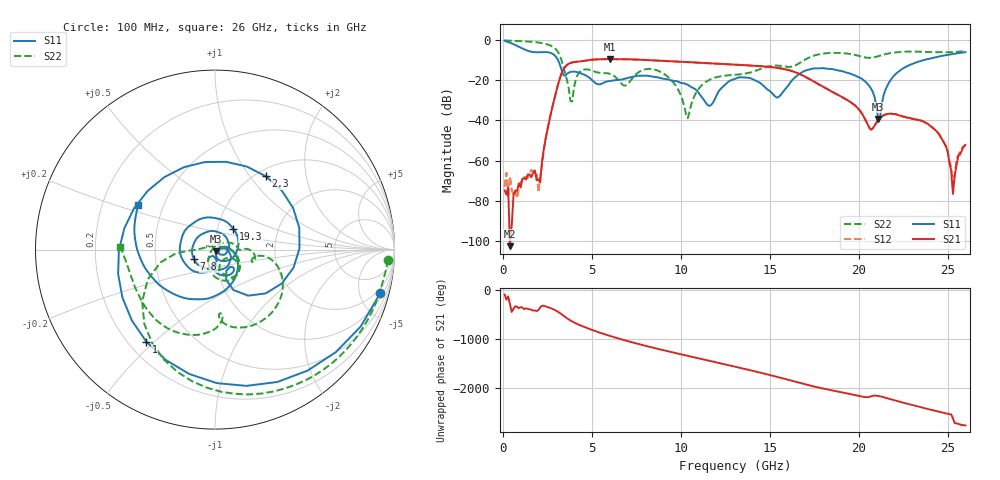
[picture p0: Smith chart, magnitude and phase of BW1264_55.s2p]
!Keysight Technologies,N5245B,MY57181159,A.13.60.06
!Date: Friday, December 18, 2020 23:54:57
!Correction: S11(Full 2 Port(1,2))
!S21(Full 2 Port(1,2))
!S12(Full 2 Port(1,2))
!S22(Full 2 Port(1,2))
!S2P File: Measurements: S11, S21, S12, S22:
# Hz S  dB  R 50
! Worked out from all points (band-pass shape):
!   260 points, 100 MHz to 26 GHz, reference 50 ohm
!   highest |S21| = -9.57 dB at 6 GHz (marker M1); lowest = -102.4 dB at 400 MHz (marker M2)
!   |S21| within 3 dB of the highest: 3.593 GHz to 13.61 GHz (10.02 GHz wide, 116 % of centre)
!   lowest |S11| = -39.3 dB at 21.1 GHz (marker M3), VSWR 1.02, Z = 50.4 - j1.01 ohm
!   |S11| at or under -10 dB: 3.1 GHz to 23.67 GHz (20.57 GHz wide, 154 % of centre)
!   |S22| runs from -38.9 to -0.3 dB; largest |S21 - S12| = 0.00055
!   S11 on the Smith chart (normalised r, x): 100 MHz: 1.43, -7.44; 1 GHz: 0.27, -0.47; 2.3 GHz: 1.11, +1.20; 7.8 GHz: 0.79, -0.09; 19.3 GHz: 1.19, +0.28; 26 GHz: 0.36, +0.23
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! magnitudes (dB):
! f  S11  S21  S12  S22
! 100 MHz  -0.4  -74.8  -72.9  -0.3
! 400 MHz  -1.4  -102.4  -67.8  -0.4
! 1 GHz  -3.9  -73.4  -71.2  -0.6
! 2 GHz  -6.2  -69.3  -75.8  -1.4
! 2.3 GHz  -6.1  -54.3  -54.9  -1.8
! 3.2 GHz  -12.1  -19.3  -19.3  -7.7
! 3.8 GHz  -15.9  -11.5  -11.5  -30.3
! 4.5 GHz  -17.0  -10.5  -10.5  -14.8
! 6 GHz  -20.5  -9.6  -9.6  -16.8
! 7.8 GHz  -17.8  -9.9  -9.9  -15.3
! 8.8 GHz  -18.9  -10.4  -10.4  -15.6
! 10.4 GHz  -22.4  -11.1  -11.1  -38.9
! 11.6 GHz  -32.8  -11.6  -11.6  -19.9
! 13.1 GHz  -19.2  -12.3  -12.3  -17.3
! 15.4 GHz  -28.7  -13.9  -13.9  -12.8
! 17.4 GHz  -14.3  -20.3  -20.3  -8.1
! 19.3 GHz  -16.2  -29.6  -29.6  -6.8
! 21.1 GHz  -39.3  -39.8  -39.9  -8.1
! 21.7 GHz  -21.3  -36.8  -36.7  -6.7
! 24.4 GHz  -8.5  -45.5  -45.7  -6.1
! 25.3 GHz  -7.0  -76.5  -71.8  -6.1
! 26 GHz  -6.1  -52.2  -52.9  -5.6
